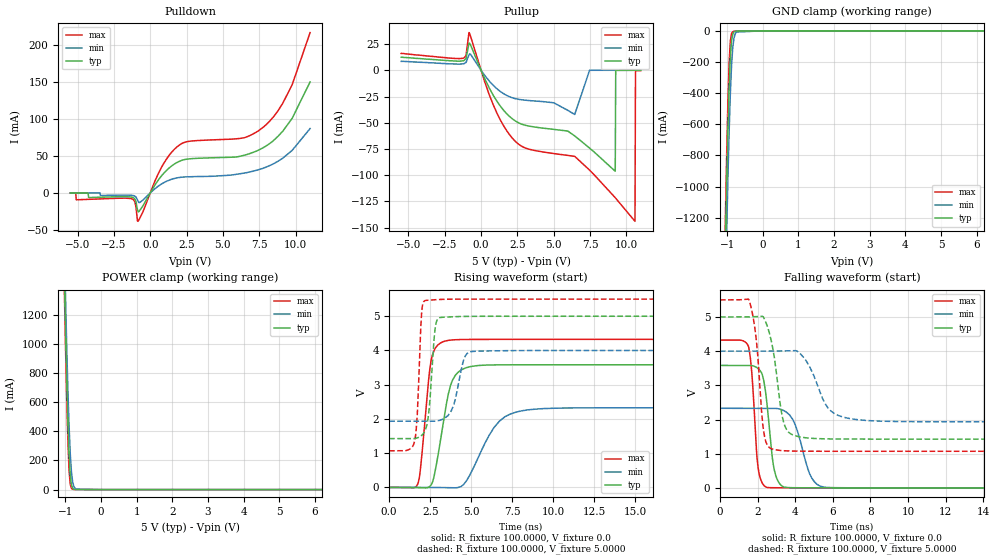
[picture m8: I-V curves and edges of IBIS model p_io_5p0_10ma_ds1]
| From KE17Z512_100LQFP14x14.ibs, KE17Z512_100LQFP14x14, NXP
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[Model] p_io_5p0_10ma_ds1
|   Model p_io_5p0_10ma_ds1
| This model was characterised for following simulation conditions:
| External (pad) voltage:
|   - Typ: 5.0V,   - Min: 4.0V,   - Max: 5.5V
| Library cells for typ/min/max conditions are connected as defined below:
|  pad - External Pad
|  ipp_do_lv - Core Input
|  ipp_obe_lv - Output Buffer Enable
|  abt_close_nor_rst_mv - vdde
|  dvdd - dvdd
|  dvss - dvss
|  esd_boost - vdde
|  ipp_dse_lv - dvdd
|  ipp_ina_280_mv - NC
|  ipp_ina_40_a_mv - NC
|  ipp_ina_40_b_mv - NC
|  ipp_ina_40_c_mv - NC
|  ipp_ina_40_d_mv - NC
|  ipp_ina_40_e_mv - NC
|  ipp_ina_40_f_mv - NC
|  ipp_ina_40_g_mv - NC
|  ipp_ina_40_h_mv - NC
|  ipp_ind_lv - NC
|  ipp_sre_lv - dvss
|  vdde - vdde
|  vsse - vsse
| All other pins connected to ground
Model_type I/O
Polarity   Non-Inverting
Enable   Active-High
Vinl =   1.5000V
Vinh =   3.5000V
Vmeas =  2.5000V
Cref =   50.0000F
C_comp   1.9155pF   1.8351pF   2.0353pF
[Model Spec]
| variable   typ   min   max
Vinh   3.5000V   2.8000V   3.8500V
Vinl   1.5000V   1.2000V   1.6500V
S_overshoot_high   5.3000V   4.3000V   5.8000V
S_overshoot_low   -0.3000V   -0.3000V   -0.3000V
Vmeas   2.5000V   2.0000V   2.7500V
[Temperature Range]   25.0000   0.1250k   -40.0000
[Voltage Range]   5.0000V   4.0000V   5.5000V
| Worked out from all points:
|   slope of the pulldown table from 0 to 0.75 V, typ, clamps not added: 33.5 ohm
|   slope of the pullup table from 0 to 0.75 V, typ, clamps not added: 34.7 ohm
|   POWER clamp passes 1 mA (typ) near -0.72 V on its own axis
|   rising waveform, R_fixture 100.0000, V_fixture 0.0: 20-80 % time 783ps typ, 1.56ns min, 503ps max; typ from 0 V to 3.58 V
|   rising waveform, R_fixture 100.0000, V_fixture 5.0000: 20-80 % time 328ps typ, 575ps min, 232ps max; typ from 1.43 V to 5 V
|   falling waveform, R_fixture 100.0000, V_fixture 0.0: 20-80 % time 416ps typ, 742ps min, 296ps max; typ from 3.58 V to 0 V
|   falling waveform, R_fixture 100.0000, V_fixture 5.0000: 20-80 % time 561ps typ, 1.01ns min, 389ps max; typ from 5 V to 1.43 V
[Pulldown]
|Voltage   I(typ)   I(min)   I(max)
-5.5V     -30uA      10uA       -300uA
-5.126V   -30uA      10uA       -400uA
-5.092V   -30uA      10uA       -9.27mA
-1.216V   -6.029mA   -3.363mA   -8.437mA
-1.046V   -8.708mA   -4.475mA   -12.87mA
-842mV    -25.16mA   -11.14mA   -38.33mA
722mV     21.75mA    11.41mA    32.62mA
1.912V    41.85mA    20.61mA    63.32mA
6.468V    50.93mA    26.8mA     74.56mA
8.202V    66.5mA     36.8mA     96.6mA
9.766V    100.8mA    57.5mA     146.2mA
11V       150mA      87mA       216.7mA
[Pullup]
|Voltage   I(typ)   I(min)   I(max)
-5.5V     12.4mA     8.5mA      16.1mA
-1.24V    9mA        6.12mA     11.45mA
-832mV    25.6mA     14.62mA    35.93mA
834mV     -23.76mA   -14.3mA    -32.79mA
2.16V     -46.33mA   -26.25mA   -64.79mA
6.444V    -62.56mA   -42.11mA   -82.04mA
7.464V    -74.1mA    -10uA      -95.08mA
9.232V    -96.21mA   10uA       -121.4mA
9.266V    -90uA      10uA       -122mA
10.59V    -30uA      0A         -143.9mA
10.63V    -30uA      0A         -410uA
11V       -40uA      -10uA      -310uA
[GND_clamp]
|Voltage   I(typ)   I(min)   I(max)
-5.5V     -66.54A    -66.41A    -66.68A
-1.08V    -1.754A    -2.051A    -1.581A
-1.046V   -1.352A    -1.659A    -1.169A
-1.012V   -977.4mA   -1.289A    -787.6mA
-978mV    -643.1mA   -949.6mA   -456.8mA
-944mV    -367.9mA   -651.2mA   -207.4mA
-910mV    -172.9mA   -405.7mA   -67.09mA
-876mV    -65.09mA   -224mA     -17.43mA
-842mV    -21.2mA    -108.6mA   -5.66mA
-740mV    -1.706mA   -8.008mA   -2.163mA
0V        -49.35pA   -428.8pA   -500.7pA
11V       0A         0A         0A
[POWER_clamp]
|Voltage   I(typ)   I(min)   I(max)
-5.5V     67.36A     67.1A      67.58A
-1.036V   1.535A     1.738A     1.426A
-1.002V   1.145A     1.361A     1.021A
-968mV    787.9mA    1.014A     654.2mA
-934mV    481mA      703.8mA    347.7mA
-900mV    245.7mA    444.9mA    136.4mA
-866mV    99.48mA    249.2mA    36.93mA
-832mV    32.56mA    121.8mA    8.258mA
-798mV    9.635mA    52.79mA    2.194mA
-696mV    574.4uA    3.321mA    568.6uA
0V        105.1pA    1.642nA    92.78pA
11V       0A         0A         0A
[Ramp]
| variable   typ   min   max
dV/dt_r  2.1495/0.7831n   1.3965/1.5612n   2.5944/0.5029n
dV/dt_f  2.1446/0.5614n   1.2403/1.0072n   2.6578/0.3885n
R_load = 100.0000
[Rising Waveform]
R_fixture= 100.0000
V_fixture= 0.0
V_fixture_min= 0.0
V_fixture_max= 0.0
|time   V(typ)   V(min)   V(max)
0s        1.046nV    12.28nV    7.831nV
1.763ns   -4.551mV   53.57uV    116.4mV
1.894ns   -6.111mV   64.72uV    473.3mV
2.554ns   64.91mV    -517.7uV   3.694V
3.408ns   2.201V     -5.86mV    4.274V
3.859ns   3.127V     -11.73mV   4.309V
4.454ns   3.446V     51.02mV    4.321V
6.717ns   3.58V      1.933V     4.324V
8.457ns   3.582V     2.265V     4.324V
40ns      3.583V     2.328V     4.324V
[Rising Waveform]
R_fixture= 100.0000
V_fixture= 5.0000
V_fixture_min= 4.0000
V_fixture_max= 5.5000
|time   V(typ)   V(min)   V(max)
0s        1.426V     1.933V     1.07V
1.57ns    1.431V     1.932V     1.38V
1.718ns   1.448V     1.931V     2.156V
1.984ns   1.519V     1.931V     5.118V
2.204ns   1.67V      1.93V      5.459V
2.444ns   2.31V      1.93V      5.471V
2.81ns    4.66V      1.937V     5.484V
3.142ns   4.965V     1.969V     5.492V
5.049ns   4.998V     3.97V      5.5V
40ns      5V         4V         5.5V
[Falling Waveform]
R_fixture= 100.0000
V_fixture= 0.0
V_fixture_min= 0.0
V_fixture_max= 0.0
|time   V(typ)   V(min)   V(max)
0s        3.583V     2.328V     4.324V
1.528ns   3.584V     2.328V     4.117V
1.697ns   3.577V     2.328V     3.336V
2.008ns   3.499V     2.328V     667.2mV
2.525ns   2.325V     2.329V     10.39mV
2.885ns   531mV      2.329V     3.095mV
3.552ns   9.478mV    2.206V     817.1uV
4.869ns   891.4uV    297.8mV    104.6uV
5.676ns   298.8uV    12.01mV    49.99uV
40ns      1.049uV    2.353uV    45.32nV
[Falling Waveform]
R_fixture= 100.0000
V_fixture= 5.0000
V_fixture_min= 4.0000
V_fixture_max= 5.5000
|time   V(typ)   V(min)   V(max)
0s        5V         4V         5.5V
1.554ns   5.001V     4V         5.478V
1.942ns   5.01V      4V         4.279V
2.316ns   4.993V     4V         1.672V
2.896ns   3.8V       4.001V     1.12V
3.455ns   1.802V     4.008V     1.085V
4.453ns   1.472V     3.812V     1.072V
5.721ns   1.432V     2.354V     1.071V
7.344ns   1.426V     1.992V     1.07V
40ns      1.426V     1.933V     1.07V
